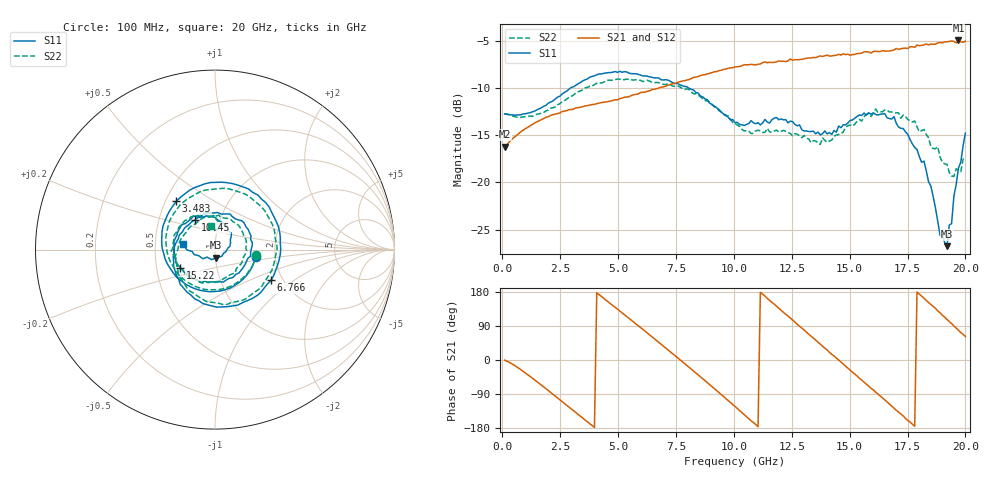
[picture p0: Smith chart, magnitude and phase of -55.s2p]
!Agilent Technologies,N5230C,MY49001569,A.09.33.09
!Agilent N5230C: A.09.33.09
!Date: Monday, July 27, 2015 20:13:03
!Correction: S11(Full 2 Port(1,2))
!S21(Full 2 Port(1,2))
!S12(Full 2 Port(1,2))
!S22(Full 2 Port(1,2))
!S2P File: Measurements: S11, S21, S12, S22:
# Hz S  dB  R 50
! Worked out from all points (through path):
!   201 points, 100 MHz to 20 GHz, reference 50 ohm
!   highest |S21| = -4.98 dB at 19.7 GHz (marker M1); lowest = -16.2 dB at 100 MHz (marker M2)
!   group delay of S21, straight-line fit = 143 ps
!   lowest |S11| = -26.8 dB at 19.2 GHz (marker M3), VSWR 1.10, Z = 50.3 - j4.6 ohm
!   |S11| at or under -10 dB: start of sweep to 2.957 GHz; 8.035 GHz to end of sweep
!   |S22| runs from -19.4 to -9.1 dB; largest |S21 - S12| = 0.017
!   S11 on the Smith chart (normalised r, x): 100 MHz: 1.58, -0.13; 3.483 GHz: 0.57, +0.35; 6.766 GHz: 1.74, -0.68; 10.45 GHz: 0.76, +0.26; 15.22 GHz: 0.66, -0.14; 20 GHz: 0.69, +0.05
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1e8  -12.74 -9.6  -16.21 -0.5  -16.19 0.0  -12.79 -7.7
1.5925e9  -12.22 -116.8  -13.49 -61.7  -13.49 -61.4  -12.76 -111.7
2.5875e9  -10.64 178.9  -12.51 -110.2  -12.53 -110.1  -11.48 -175.9
3.483e9  -9.24 128.8  -11.97 -153.7  -12.00 -154.0  -10.20 133.0
4.876e9  -8.27 61.2  -11.26 139.1  -11.27 138.8  -9.12 64.9
5.871e9  -8.57 14.5  -10.65 90.6  -10.63 90.6  -9.16 19.9
6.7665e9  -8.97 -28.7  -10.01 46.2  -10.02 46.3  -9.46 -20.5
8.3585e9  -10.49 -107.6  -8.87 -34.0  -8.82 -33.8  -10.63 -96.8
9.254e9  -12.08 -158.1  -8.28 -80.6  -8.26 -80.5  -12.06 -142.4
1.005e10  -13.68 151.4  -7.78 -122.6  -7.82 -122.6  -13.78 172.8
1.0448e10  -13.98 123.8  -7.56 -144.0  -7.64 -144.2  -14.56 147.5
1.17415e10  -13.21 48.3  -7.30 147.5  -7.25 146.7  -14.56 68.6
1.2637e10  -13.87 1.3  -7.02 100.2  -7.02 99.6  -14.84 19.3
1.3433e10  -14.59 -44.3  -6.78 58.0  -6.80 57.8  -15.59 -24.8
1.45275e10  -14.04 -112.2  -6.44 -0.1  -6.47 0.2  -14.93 -88.3
1.5224e10  -13.21 -152.8  -6.46 -37.3  -6.41 -37.3  -13.84 -130.1
1.59205e10  -12.80 174.8  -6.32 -74.4  -6.08 -74.1  -13.03 -168.0
1.67165e10  -13.25 134.4  -6.10 -116.1  -6.03 -115.7  -12.56 155.7
1.79105e10  -16.52 64.0  -5.47 179.5  -5.59 179.5  -14.13 103.7
1.9204e10  -26.76 -84.2  -5.12 107.3  -5.22 107.6  -18.09 80.1
1.97015e10  -18.48 -166.5  -4.98 78.5  -5.15 78.7  -18.69 97.4
2e10  -14.79 169.9  -5.06 62.0  -5.16 61.5  -17.38 100.2
